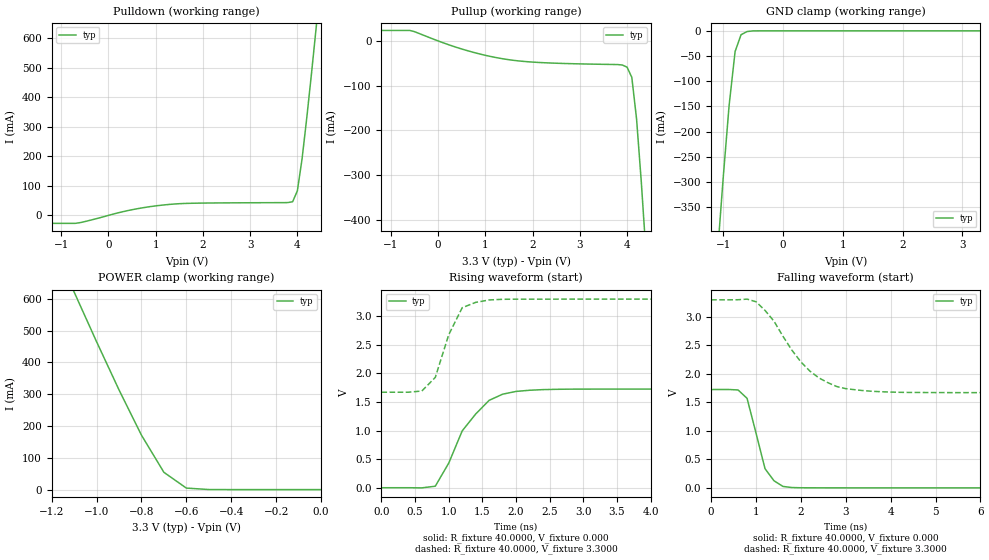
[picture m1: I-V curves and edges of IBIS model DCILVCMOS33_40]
| / 7\'7
| \ \   Xilinx Inc.
| / /
| \_\/.\   IBIS Model for Virtex-II
[IBIS ver]   2.1
[File name]   dci3340.ibs
[File Rev]   1.1
[Date]   Aug. 02, 2001
[Source]   Hspice simulations (08-02: TT, SS, FF)
[Notes]   Xilinx IBIS model for LVDCI 3.3V 40 ohms driver
[Disclaimer] The data in this model is derived from SPICE simulations using
   modeling information extracted from the target process. While
   a great deal of care has been taken to provide information
   that is accurate, this model is considered preliminary as it
   has not been verified by actual silicon measurement. Treat the
   data in this model as preliminary until actual silicon
   verification is performed.
[Copyright]   Copyright 2001, Xilinx Inc., All rights reserved
|   Component Virtex_II
[Component]   Virtex_II
[Manufacturer]   Xilinx Inc.
[Package]
| variable   typ   min   max
R_pkg   0.1000   NA   NA
L_pkg   0.8000nH   NA   NA
C_pkg   0.5000pF   NA   NA
[Pin]  signal_name   model_name   R_pin   L_pin   C_pin
io   DCILVCMOS33_40   DCILVCMOS33_40
| ins  insig   inp
| ens  ensig   inp
PGND   GND   GND
VCCO   VCCO   POWER
| Models and submodels in the file (1): DCILVCMOS33_40 (I/O)
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|   Model DCILVCMOS33_40
[Model]   DCILVCMOS33_40
Model_type   I/O
Polarity   Non-Inverting
Enable   Active-Low
Vinh = 2.0V
Vinl = 0.8V
Vmeas =   1.4000V
Cref =  35.0000pF
Rref =   1.0000M
Vref =  0.000V
C_comp   7.0000pF   NA   NA
[Temperature Range]   25.0000   NA   NA
[Voltage Range]   3.3000V   NA   NA
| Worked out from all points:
|   slope of the pulldown table from 0 to 0.495 V, typ, clamps not added: 26 ohm
|   slope of the pullup table from 0 to 0.495 V, typ, clamps not added: 27.6 ohm
|   GND clamp passes 1 mA (typ) near -0.57 V on its own axis
|   POWER clamp passes 1 mA (typ) near -0.52 V on its own axis
|   rising waveform, R_fixture 40.0000, V_fixture 0.000: 20-80 % time 519ps typ, NA min, NA max; typ from 0 V to 1.73 V
|   rising waveform, R_fixture 40.0000, V_fixture 3.3000: 20-80 % time 308ps typ, NA min, NA max; typ from 1.67 V to 3.3 V
|   falling waveform, R_fixture 40.0000, V_fixture 0.000: 20-80 % time 335ps typ, NA min, NA max; typ from 1.73 V to 0 V
|   falling waveform, R_fixture 40.0000, V_fixture 3.3000: 20-80 % time 940ps typ, NA min, NA max; typ from 3.3 V to 1.67 V
[Pulldown]
| voltage   I(typ)   I(min)   I(max)
-3.3V     -26.92mA   NA         NA
-700mV    -26.92mA   NA         NA
500mV     19.2mA     NA         NA
1.2V      35.85mA    NA         NA
1.7V      40.85mA    NA         NA
3.9V      46.25mA    NA         NA
4V        83.11mA    NA         NA
4.1V      192mA      NA         NA
4.2V      331.6mA    NA         NA
4.3V      481.9mA    NA         NA
4.5V      796.2mA    NA         NA
6.6V      4.268A     NA         NA
[Pullup]
| voltage   I(typ)   I(min)   I(max)
-3.3V     23.49mA    NA         NA
-600mV    23.49mA    NA         NA
500mV     -18.08mA   NA         NA
1.4V      -40.51mA   NA         NA
2.2V      -48.62mA   NA         NA
3.9V      -53.96mA   NA         NA
4V        -58.78mA   NA         NA
4.1V      -81.59mA   NA         NA
4.2V      -174mA     NA         NA
4.3V      -314.4mA   NA         NA
4.5V      -635mA     NA         NA
6.6V      -4.317A    NA         NA
[GND_clamp]
| voltage   I(typ)   I(min)   I(max)
-3.3V     -4.301A    NA         NA
-1.1V     -452.1mA   NA         NA
-1V       -293.4mA   NA         NA
-900mV    -148.1mA   NA         NA
-800mV    -41.07mA   NA         NA
-700mV    -7.668mA   NA         NA
-600mV    -1.449mA   NA         NA
-400mV    -8.141uA   NA         NA
3.3V      540.8nA    NA         NA
[POWER_clamp]
| voltage   I(typ)   I(min)   I(max)
-3.3V     4.254A     NA         NA
-1.1V     621.4mA    NA         NA
-1V       465.1mA    NA         NA
-900mV    313.6mA    NA         NA
-800mV    171.2mA    NA         NA
-700mV    54.37mA    NA         NA
-600mV    4.797mA    NA         NA
-500mV    289.2uA    NA         NA
0V        540.8nA    NA         NA
[Ramp]
| variable   typ   min   max
dV/dt_r   1.0356/0.4397n   NA   NA
dV/dt_f   0.9774/0.9182n   NA   NA
R_load = 40.0000
[Rising Waveform]
R_fixture = 40.0000
V_fixture = 0.000
| time   V(typ)   V(min)   V(max)
0s        10.36uV    NA         NA
800ps     26.21mV    NA         NA
1ns       431.1mV    NA         NA
1.2ns     994.9mV    NA         NA
1.4ns     1.29V      NA         NA
1.6ns     1.529V     NA         NA
1.8ns     1.637V     NA         NA
2ns       1.685V     NA         NA
2.8ns     1.725V     NA         NA
10ns      1.726V     NA         NA
[Rising Waveform]
R_fixture = 40.0000
V_fixture = 3.3000
V_fixture_min = 3.0000
V_fixture_max = 3.6000
| time   V(typ)   V(min)   V(max)
0s        1.671V     NA         NA
400ps     1.671V     NA         NA
600ps     1.692V     NA         NA
800ps     1.93V      NA         NA
1ns       2.678V     NA         NA
1.2ns     3.15V      NA         NA
1.4ns     3.244V     NA         NA
1.6ns     3.285V     NA         NA
2ns       3.299V     NA         NA
10ns      3.3V       NA         NA
[Falling Waveform]
R_fixture = 40.0000
V_fixture = 0.000
| time   V(typ)   V(min)   V(max)
0s        1.726V     NA         NA
600ps     1.718V     NA         NA
800ps     1.571V     NA         NA
1ns       959.9mV    NA         NA
1.2ns     336.5mV    NA         NA
1.4ns     124.5mV    NA         NA
1.6ns     25.14mV    NA         NA
1.8ns     5.577mV    NA         NA
2.2ns     1.174mV    NA         NA
10ns      2.961uV    NA         NA
[Falling Waveform]
R_fixture = 40.0000
V_fixture = 3.3000
V_fixture_min = 3.0000
V_fixture_max = 3.6000
| time   V(typ)   V(min)   V(max)
0s        3.3V       NA         NA
800ps     3.312V     NA         NA
1ns       3.266V     NA         NA
1.4ns     2.925V     NA         NA
1.8ns     2.415V     NA         NA
2.2ns     2.049V     NA         NA
2.6ns     1.846V     NA         NA
3ns       1.741V     NA         NA
4.4ns     1.675V     NA         NA
10ns      1.671V     NA         NA
